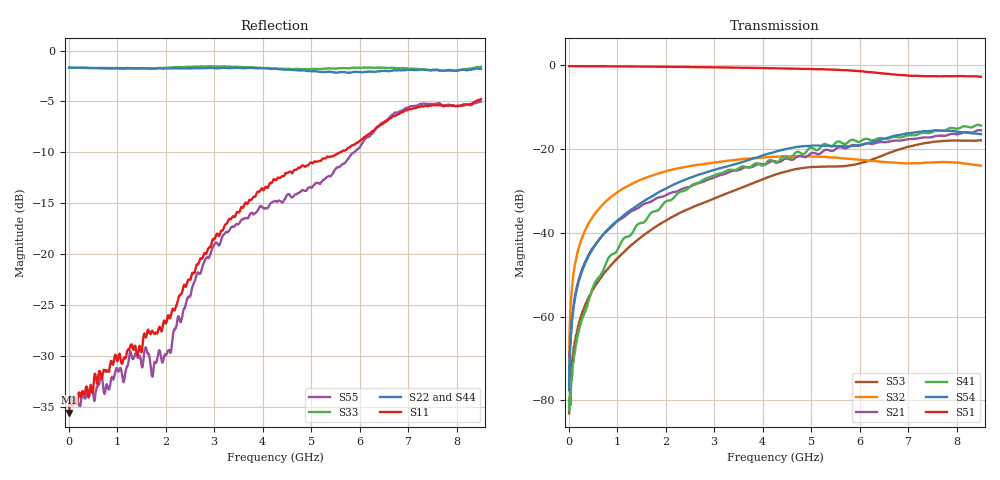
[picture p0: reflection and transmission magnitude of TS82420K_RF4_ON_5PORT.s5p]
!Created with skrf (http://scikit-rf.org).
# GHz S RI R 50.0
!freq ReS11 ImS11 ReS12 ImS12 ReS13 ImS13
! ReS14 ImS14 ReS15 ImS15
! ReS21 ImS21 ReS22 ImS22 ReS23 ImS23
! ReS24 ImS24 ReS25 ImS25
! ReS31 ImS31 ReS32 ImS32 ReS33 ImS33
! ReS34 ImS34 ReS35 ImS35
! ReS41 ImS41 ReS42 ImS42 ReS43 ImS43
! ReS44 ImS44 ReS45 ImS45
! ReS51 ImS51 ReS52 ImS52 ReS53 ImS53
! ReS54 ImS54 ReS55 ImS55
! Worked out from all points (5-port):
!   1601 points, 10 MHz to 8.5 GHz, reference 50 ohm
!   strongest paths, dB at 10 MHz, 2.132 GHz, 4.255 GHz, 6.378 GHz, 8.5 GHz:
!     S51: -0.2, -0.4, -0.7, -1.8, -2.8
!     S54: -77.6, -28.7, -20.7, -17.9, -16.4
!     S41: -82.1, -32.0, -23.2, -17.4, -14.4
!     S21: -75.9, -30.4, -22.9, -18.4, -15.5
!     S32: -69.6, -24.9, -21.9, -22.9, -24.0
!     S53: -83.1, -36.2, -26.1, -22.0, -17.9
!   lowest |S11| = -35.6 dB at 10 MHz (marker M1), VSWR 1.03, Z = 51.7 + j0.0341 ohm
!   |S11| at or under -10 dB: start of sweep to 5.598 GHz
